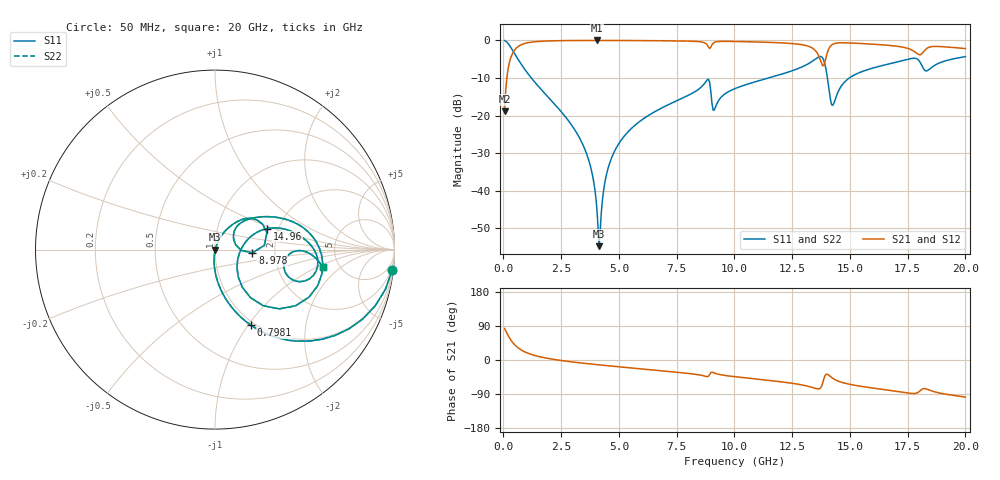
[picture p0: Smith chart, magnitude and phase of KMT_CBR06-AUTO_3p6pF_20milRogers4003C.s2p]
! Data measured by Modelithics Inc. support@modelithics.com 813-866-6335
! KEMET CBR06-AUTO 3.6pF, Pad Width= 0.851mm, Pad Length= 0.64mm, Pad Gap= 0.62mm, 20mil Rogers 4003C substrate Data, January 2022
# hz S ma R 50
! 2 Port Network Data from SP1.SP block
! freq  magS11  angS11  magS21  angS21  magS12  angS12  magS22  angS22
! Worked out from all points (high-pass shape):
!   401 points, 50 MHz to 20 GHz, reference 50 ohm
!   highest |S21| = -0.02 dB at 4.04 GHz (marker M1); lowest = -18.9 dB at 50 MHz (marker M2)
!   |S21| within 3 dB of the highest: 434.9 MHz to 13.54 GHz (13.11 GHz wide, 188 % of centre); 14.04 GHz to 17.8 GHz (3.764 GHz wide, 23.6 % of centre)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
!   lowest |S11| = -54.8 dB at 4.14 GHz (marker M3), VSWR 1.00, Z = 50.2 - j0.0714 ohm
!   |S11| at or under -10 dB: 1.207 GHz to 11.47 GHz (10.27 GHz wide, 162 % of centre); 14.03 GHz to 14.97 GHz (949.5 MHz wide, 6.55 % of centre)
!   |S22| runs from -54.8 to -0.1 dB; largest |S21 - S12| = 0
!   S11 on the Smith chart (normalised r, x): 50 MHz: 1, -17; 798.1 MHz: 0.96, -1.03; 8.978 GHz: 1.52, -0.06; 14.96 GHz: 1.75, +0.46; 20 GHz: 3.73, -1.14
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5e7  0.9935 -6.7  0.1133 83.3  0.1133 83.3  0.9935 -6.7
2.99375e8  0.8241 -35.4  0.5656 54.6  0.5656 54.6  0.8241 -35.4
7.98125e8  0.4678 -64.5  0.8829 25.4  0.8829 25.4  0.4678 -64.5
3.391625e9  0.04396 -95.9  0.9973 -8.0  0.9973 -8.0  0.04396 -95.9
3.8405e9  0.01688 -95.1  0.998 -11.0  0.998 -11.0  0.01688 -95.1
4.04e9  0.005964 -84.9  0.9981 -12.2  0.9981 -12.2  0.005964 -84.9
4.13975e9  0.001826 -22.9  0.9981 -12.8  0.9981 -12.8  0.001826 -22.9
4.439e9  0.01532 68.4  0.9979 -14.7  0.9979 -14.7  0.01532 68.4
4.838e9  0.03486 69.8  0.9973 -17.0  0.9973 -17.0  0.03486 69.8
6.73325e9  0.1207 61.0  0.9899 -27.8  0.9899 -27.8  0.1207 61.0
8.828e9  0.3008 28.1  0.8648 -43.9  0.8648 -43.9  0.3008 28.1
8.977625e9  0.209 -5.0  0.8108 -33.4  0.8108 -33.4  0.209 -5.0
9.12725e9  0.1185 28.7  0.94 -34.2  0.94 -34.2  0.1185 28.7
1.0025e10  0.2283 44.5  0.9673 -44.0  0.9673 -44.0  0.2283 44.5
1.336662e10  0.5259 11.2  0.793 -72.4  0.793 -72.4  0.5259 11.2
1.371575e10  0.6107 -12.9  0.5518 -74.4  0.5518 -74.4  0.6107 -12.9
1.391525e10  0.4872 -42.7  0.5123 -42.3  0.5123 -42.3  0.4872 -42.7
1.426438e10  0.1371 -9.1  0.8899 -48.5  0.8899 -48.5  0.1371 -9.1
1.496262e10  0.3144 21.9  0.9258 -63.9  0.9258 -63.9  0.3144 21.9
1.670825e10  0.4877 8.3  0.8571 -79.9  0.8571 -79.9  0.4877 8.3
1.8005e10  0.5315 -19.2  0.6436 -83.0  0.6436 -83.0  0.5315 -19.2
2e10  0.6077 -9.1  0.779 -97.7  0.779 -97.7  0.6077 -9.1
